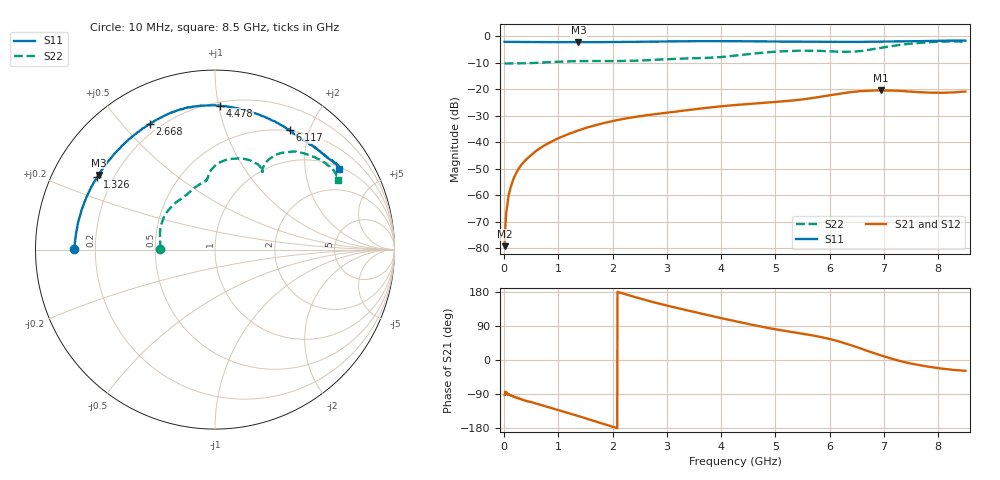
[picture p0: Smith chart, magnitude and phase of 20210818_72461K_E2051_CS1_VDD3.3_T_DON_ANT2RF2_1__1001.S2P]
!Agilent Technologies,E5071C,MY46417908,A.11.23
!Date: Wed Aug 18 14:27:18 2021
!Data & Calibration Information:
!Freq	S11:SOLT2(ON)	S21:SOLT2(ON)	S12:SOLT2(ON)	S22:SOLT2(ON)
!PortZ  Port1:50+j0  Port2:50+j0
!Above PortZ is port z conversion or system Z0 setting when saving the data.
!When reading, reference impedance value at option line is always used.
# Hz S dB R 50
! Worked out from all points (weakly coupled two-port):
!   1601 points, 10 MHz to 8.5 GHz, reference 50 ohm
!   highest |S21| = -20.42 dB at 6.94 GHz (marker M1); lowest = -79.2 dB at 10 MHz (marker M2)
!   lowest |S11| = -2.3 dB at 1.368 GHz (marker M3), VSWR 7.70, Z = 7.04 + j14.4 ohm
!   |S11| at or under -10 dB: nowhere
!   |S22| runs from -10.3 to -2.0 dB; largest |S21 - S12| = 0.0004
!   S11 on the Smith chart (normalised r, x): 10 MHz: 0.12, +0.00; 1.326 GHz: 0.14, +0.28; 2.668 GHz: 0.16, +0.60; 4.478 GHz: 0.23, +1.01; 6.117 GHz: 0.49, +1.70; 8.5 GHz: 1.07, +3.02
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1e7  -2.10 179.7  -79.16 -92.7  -79.47 -80.4  -10.27 179.7
6.30625e7  -2.14 178.5  -62.69 -88.4  -62.77 -89.8  -10.29 178.5
1.055125e8  -2.14 177.6  -58.21 -92.6  -58.21 -92.4  -10.30 177.5
1.851062e8  -2.16 175.7  -53.21 -96.8  -53.25 -96.7  -10.30 175.6
3.018438e8  -2.18 173.0  -49.07 -102.8  -48.93 -102.6  -10.26 173.2
5.087875e8  -2.20 168.3  -44.61 -111.4  -44.61 -111.2  -10.13 168.7
7.051188e8  -2.21 163.5  -41.66 -119.8  -41.68 -119.7  -9.92 163.7
1.32595e9  -2.26 148.4  -35.84 -146.1  -35.85 -146.1  -9.40 145.1
1.3684e9  -2.27 147.4  -35.54 -147.9  -35.54 -147.8  -9.39 143.8
1.426769e9  -2.25 145.8  -35.12 -150.4  -35.12 -150.4  -9.38 141.9
2.668431e9  -2.07 117.3  -29.69 155.9  -29.69 155.8  -9.04 111.8
2.843538e9  -2.01 114.1  -29.24 149.3  -29.24 149.2  -8.82 108.5
4.255e9  -1.89 91.7  -25.96 102.3  -25.97 102.3  -7.36 93.9
4.477862e9  -1.92 87.9  -25.60 95.6  -25.60 95.7  -6.84 91.5
5.066856e9  -2.02 76.6  -24.66 79.5  -24.67 79.6  -5.77 79.3
5.671769e9  -2.08 65.0  -23.33 65.2  -23.34 65.3  -5.48 65.0
6.117494e9  -2.11 57.9  -21.87 51.1  -21.90 51.2  -5.79 59.1
6.939962e9  -2.04 47.8  -20.42 12.2  -20.45 12.2  -4.42 58.5
7.088538e9  -1.99 46.4  -20.46 5.8  -20.48 5.6  -3.91 56.7
7.444056e9  -1.93 42.6  -20.84 -7.6  -20.84 -7.6  -2.95 49.8
7.937538e9  -1.73 37.3  -21.30 -20.2  -21.29 -20.2  -2.14 38.0
8.5e9  -1.67 33.1  -20.88 -28.5  -20.89 -28.7  -2.10 29.6
